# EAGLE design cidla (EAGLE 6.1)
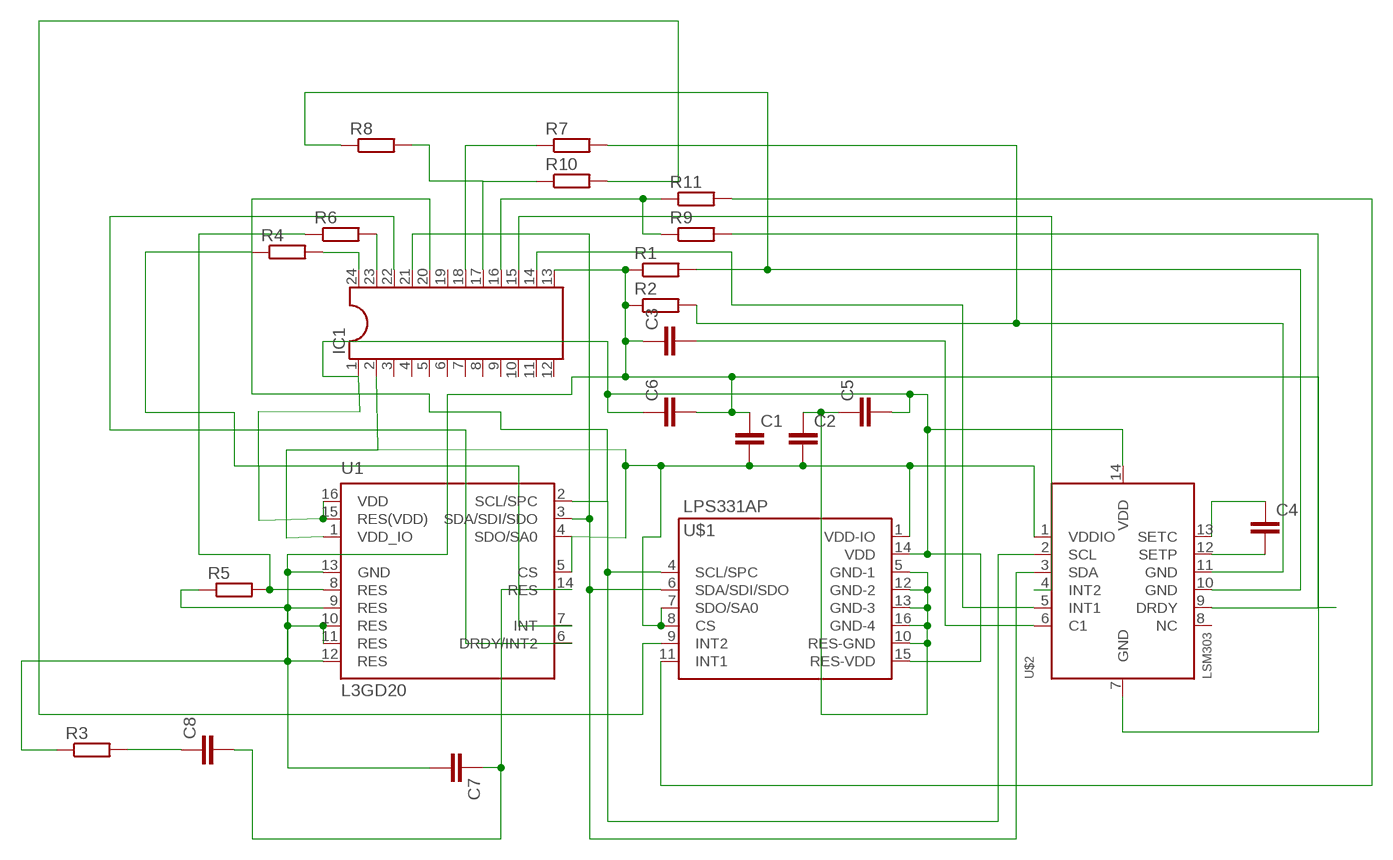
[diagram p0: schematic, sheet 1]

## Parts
C1  C-EUC0402  [C0402]
C2  C-EUC0402  [C0402]
C3  C-EUC0402  [C0402]
C4  C-EUC0402  [C0402]
C5  C-EUC0402  [C0402]
C6  C-EUC0402  [C0402]
C7  C-EUC0402  [C0402]
C8  C-EUC0402  [C0402]
IC1  DIL24-6  [DIL24-6]
R1  R-EU_R0402  [R0402]
R2  R-EU_R0402  [R0402]
R3  R-EU_R0402  [R0402]
R4  R-EU_R0402  [R0402]
R5  R-EU_R0402  [R0402]
R6  R-EU_R0402  [R0402]
R7  R-EU_R0402  [R0402]
R8  R-EU_R0402  [R0402]
R9  R-EU_R0402  [R0402]
R10  R-EU_R0402  [R0402]
R11  R-EU_R0402  [R0402]
U1  L3GD20  [LGA-16L]
U$1  LPS331AP  [HCLGA-16L]
U$2  LSM303  [LGA14]

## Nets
N$1: C5.2 C6.1 IC1.1 U1.15(RES(VDD)) U1.16(VDD) U$1.14(VDD) U$1.15(RES-VDD) U$2.14(VDD)
N$2: C1.2 C2.2 IC1.2 U1.1(VDD_IO) U1.4(SDO/SA0) U1.5(CS) U$1.1(VDD-IO) U$1.7(SDO/SA0) U$1.8(CS) U$2.1(VDDIO)
N$3: C1.1 C3.1 C6.2 C7.2 IC1.13 R1.1 R2.1 R3.1 R5.1 U1.9(RES) U1.10(RES) U1.11(RES) U1.12(RES) U1.13(GND) U$2.7(GND)
N$4: IC1.24 R4.2
N$5: IC1.23 R6.2
N$6: IC1.17 R8.2 R10.1
N$7: IC1.18 R7.1
N$8: IC1.16 R9.1 R11.1
N$9: IC1.14 U$2.5(INT1)
N$10: C3.2 U$2.6(C1)
N$12: R11.2 U$1.11(INT1)
N$14: C2.1 C5.1 U$1.5(GND-1) U$1.10(RES-GND) U$1.12(GND-2) U$1.13(GND-3) U$1.16(GND-4)
N$16: R10.2 U$1.9(INT2)
N$17: R1.2 R8.1 U$2.10(GND)
N$18: C4.2 U$2.12(SETP)
N$19: C4.1 U$2.13(SETC)
N$20: R2.2 R7.2 U$2.11(GND)
N$21: IC1.15 U$2.4(INT2)
N$22: IC1.21 U1.3(SDA/SDI/SDO) U$1.6(SDA/SDI/SDO) U$2.3(SDA)
N$23: IC1.20 U1.2(SCL/SPC) U$1.4(SCL/SPC) U$2.2(SCL)
N$24: R4.1 U1.7(INT)
N$25: C7.1 C8.2 U1.14(RES)
N$26: R5.2 R6.1 U1.8(RES)
N$27: IC1.22 U1.6(DRDY/INT2)
N$28: C8.1 R3.2
N$29: R9.2 U$2.9(DRDY)
Unconnected: IC1.3 IC1.4 IC1.5 IC1.6 IC1.7 IC1.8 IC1.9 IC1.10 IC1.11 IC1.12 IC1.19 U$2.8(NC)

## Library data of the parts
C1-C8 = rcl:C-EU: CAPACITOR, European symbol
IC1 = ic-package:DIL24: Dual In Line
R1-R11 = rcl:R-EU_: RESISTOR, European symbol
U1 = cansat_jecnaci:L3GD20: L3GD20 MEMS motion sensor - three-axis digital output gyroscope
U$1 = cansat_jecnaci:LPS331AP: LPS331AP MEMS pressure sensor: 260-1260 mbar absolute digital output barometer Features ? 260 to 1260 mbar absolute pressure range ? High-resolution mode: 0.020 mbar RMS ? Low power consumption: ? Low resolution mode: 5.5 ?A ? High resolution mode: 30 ?A ? High overpressure capability: 20x full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
U$2 = LSM303:LSM303

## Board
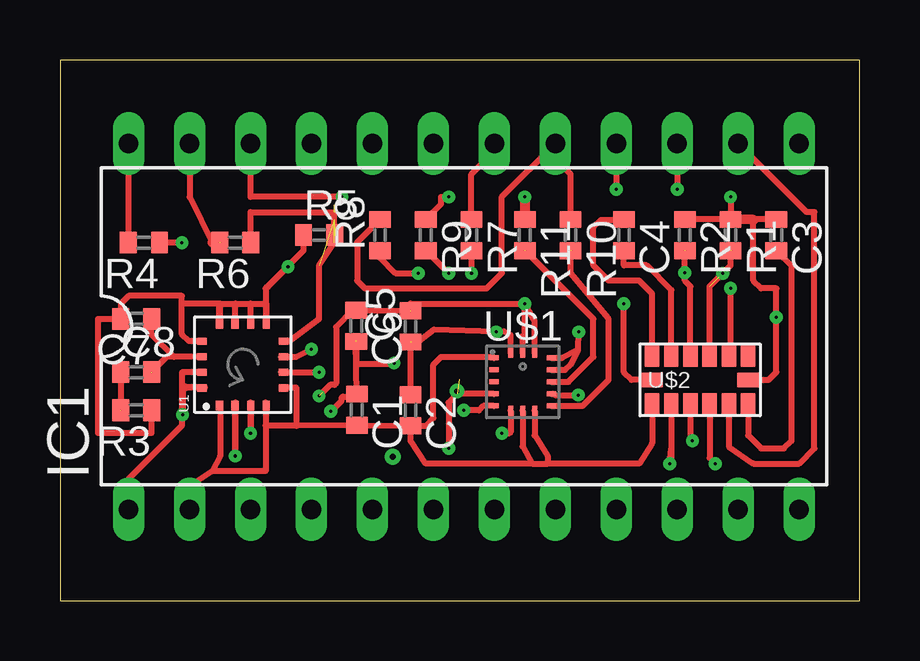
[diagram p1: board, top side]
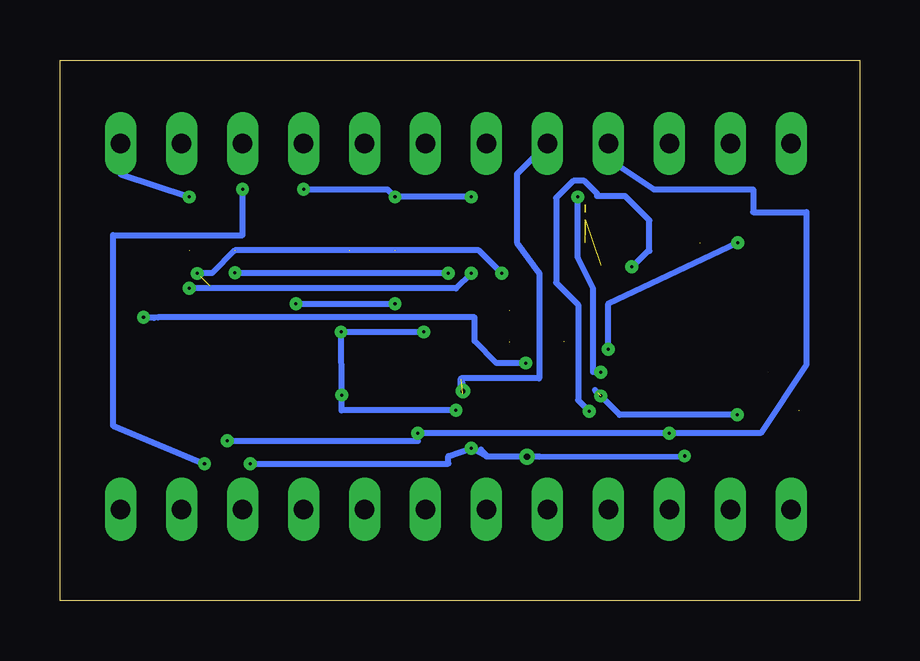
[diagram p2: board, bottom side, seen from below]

Size 33.33 x 22.53 mm. Coordinates in mm from the lower left corner, seen from the top.
Outline: 0,0 33.33,0 33.33,22.53 0,22.53 0,0
Copper layers (1*16): Top 0.035mm / dielectric 1.5mm / Bottom 0.035mm
Design rules "default": minimum track width 10mil, minimum drill 24mil, track to track 8mil, track to pad 8mil, pad to pad 8mil, via to via 8mil, smd to smd 8mil, copper to edge 40mil, drill to drill 8mil, minimum pad ring 10mil, minimum via ring 8mil, stop-mask expansion 4mil, vias tented up to drill 0mil, thermal gap 10mil

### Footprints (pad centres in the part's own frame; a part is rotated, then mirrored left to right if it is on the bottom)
C0402 = smd 0.7 x 0.9: 1 -0.65,0; 2 0.65,0
DIL24-6 = drill 0.813 long: 1 -13.97,-7.62; 2 -11.43,-7.62; 3 -8.89,-7.62; 4 -6.35,-7.62; 5 -3.81,-7.62; 6 -1.27,-7.62; 7 1.27,-7.62; 8 3.81,-7.62; 9 6.35,-7.62; 10 8.89,-7.62; 11 11.43,-7.62; 12 13.97,-7.62; 13 13.97,7.62; 14 11.43,7.62; 15 8.89,7.62; 16 6.35,7.62; 17 3.81,7.62; 18 1.27,7.62; 19 -1.27,7.62; 20 -3.81,7.62; 21 -6.35,7.62; 22 -8.89,7.62; 23 -11.43,7.62; 24 -13.97,7.62
R0402 = smd 0.7 x 0.9: 1 -0.65,0; 2 0.65,0
LGA-16L = smd 0.4 x 0.3: 1 -1.7,0.975; 2 -1.7,0.325; 3 -1.7,-0.325; 4 -1.7,-0.975; 9 1.7,-0.975; 10 1.7,-0.325; 11 1.7,0.325; 12 1.7,0.975 | smd 0.3 x 0.4: 5 -0.975,-1.7; 6 -0.325,-1.7; 7 0.325,-1.7; 8 0.975,-1.7; 13 0.975,1.7; 14 0.325,1.7; 15 -0.325,1.7; 16 -0.975,1.7
HCLGA-16L = smd 0.406 x 0.203: 1 0.3,2.5; 2 0.3,2; 3 0.3,1.5; 4 0.3,1; 5 0.3,0.5; 9 2.7,0.5; 10 2.7,1; 11 2.7,1.5; 12 2.7,2; 13 2.7,2.5 | smd 0.203 x 0.406: 6 1,0.3; 7 1.5,0.3; 8 2,0.3; 14 2,2.7; 15 1.5,2.7; 16 1,2.7
LGA14 = smd 0.9 x 0.6: 1 1,-2; 2 1,-1.2; 3 1,-0.4; 4 1,0.4; 5 1,1.2; 6 1,2; 8 -1,2; 9 -1,1.2; 10 -1,0.4; 11 -1,-0.4; 12 -1,-1.2; 13 -1,-2 | smd 0.6 x 0.9: 7 0,2; 14 0,-2

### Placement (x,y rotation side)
C1  12.37,7.96 270 top
C2  14.61,7.94 270 top
C3  29.84,15.24 270 top
C4  23.5,15.24 270 top
C5  14.61,11.43 90 top
C6  12.34,11.46 270 top
C7  3.17,11.75 180 top
C8  3.17,9.53 0 top
IC1  16.83,11.43 0 top
R1  27.94,15.24 270 top
R2  26.04,15.24 270 top
R3  3.17,7.94 180 top
R4  3.49,14.92 180 top
R5  10.79,15.24 0 top
R6  7.3,14.92 180 top
R7  17.14,15.24 270 top
R8  13.34,15.24 90 top
R9  15.24,15.24 270 top
R10  21.27,15.24 270 top
R11  19.37,15.24 270 top
U1  7.62,9.84 90 top
U$1  17.78,7.62 0 top
U$2  26.67,9.21 270 top

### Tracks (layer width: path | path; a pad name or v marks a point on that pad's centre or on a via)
N$1  (via drill 0.13)  (2 unrouted)
  Top 0.254: U1.15 5.08,9.52 5.08,9.07 | 5.08,9.07 5.08,8.89 5.11,8.89 | IC1.1 2.86,5.08 5.08,7.3 5.08,8.87 U1.16 5.28,8.87 5.08,9.07 | v19.37,12.38 14.61,12.38 14.59,12.08 C6.1 12.21,12.11 11.51,11.4 11.51,9.07 11.43,8.99 11.25,8.99 v10.79,8.53 | v19.37,12.38 19.37,11.11 19.28,11.03 U$1.15 | U$1.14 19.78,11.65 19.58,12.01 v19.37,12.38 | U$2.14 23.81,9.21 23.5,9.53 v23.5,12.38 | 6.03,8.89 5.11,8.89 | 5.11,8.89 5.11,8.91 | 5.11,8.89 v5.11,7.75
  Bottom 0.254: v23.5,12.38 v19.37,12.38 | v5.11,7.75 10.01,7.75 v10.79,8.53 10.92,8.66 11.04,8.78
N$2
  Top 0.254: U1.1 6.67,8.12 6.67,6.03 6.35,5.4 | 6.35,5.4 5.4,4.76 IC1.2 | 8.57,8.12 U1.4 8.57,8.16 | 8.57,8.12 8.57,7.3 | 8.57,7.3 8.57,5.4 6.35,5.4 | U1.5 9.34,8.89 9.84,8.89 9.84,7.3 | 9.84,7.3 8.57,7.3 | 8.57,8.12 8.57,8.16 | 8.57,8.16 8.57,8.26 | 19.68,5.71 20.32,5.71 | U$1.8 19.78,6.89 20.32,6.03 20.32,5.71 | U$2.1 24.67,6.57 24.13,5.71 20.32,5.71 | 14.61,7.3 14.59,7.29 C1.2 9.86,7.29 9.84,7.3 | 14.61,7.3 C2.2 14.61,6.67 15.24,5.71 19.68,5.71 | 14.61,7.3 15.24,7.3 15.56,7.62 15.56,9.84 15.88,10.16 18.04,10.16 U$1.1 | U$1.7 19.28,6.44 19.68,5.71
N$3  (via drill 0.13)  (1 unrouted)
  Top 0.254: 6.67,12.38 6.67,11.56 U1.12 6.64,12.36 6.67,12.38 | 6.67,12.38 7.3,12.38 | 7.3,12.38 7.94,12.38 | 7.94,12.38 8.57,12.38 | 8.57,12.38 8.6,12.36 U1.9 8.6,13.06 8.61,13.08 8.66,13.08 v9.5,13.92 | U1.10 7.94,11.55 7.94,12.38 | U1.11 7.3,11.55 7.3,12.38 | U1.13 5.38,10.82 5.08,11.11 5.08,12.38 | 5.08,12.38 5.08,12.7 2.86,12.7 2.54,12.38 2.54,11.76 C7.2 1.59,11.75 1.59,6.99 3.81,6.99 R3.1 | 6.67,12.38 5.08,12.38 | R5.1 10.14,14.59 8.57,13.02 8.57,12.38 | 12.32,10.82 C1.1 12.27,8.51 11.79,8.51 11.73,8.46 11.73,8.33 11.3,7.9 v11.28,7.9 | C3.1 R1.1 | R1.1 R2.1 | v27.94,16.83 R1.1 | U$2.7 29.53,9.21 29.84,9.53 v29.84,11.81 29.84,13.02 29.21,13.02 28.89,13.34 28.89,15.88 | C6.2 12.34,9.91 12.37,9.88 13.89,9.88 v13.92,9.91
  Top 0.406: 27.94,15.88 27.95,15.89 R1.1 28.89,15.88
  Bottom 0.254: v27.94,16.83 30.8,17.78 IC1.13 | v13.92,9.91 15.14,9.91 16.05,10.82 16.05,11.81 29.23,11.81 29.41,11.79 29.82,11.79 v29.84,11.81 | v9.5,13.92 9.47,13.92 8.81,14.58 8.76,14.58 8.76,15.85 9.78,16.87 10.95,16.87 10.95,16.97 11.48,17.5 11.94,17.5 12.65,16.79 12.65,13.26 11.73,12.34 11.73,8.36 v11.28,7.9
N$4
  Top 0.254: 2.86,14.92 IC1.24
  Top 0.406: R4.2 2.86,14.92
N$5  (1 unrouted)
  Top 0.254: IC1.23 5.4,16.83 6.35,14.92
  Top 0.406: 6.35,14.92 6.67,14.92
N$6
  Top 0.254: R10.1 21.27,17.78 20.64,18.41 IC1.17 18.41,16.83 18.41,13.65 17.78,13.02 12.7,13.02 12.38,13.34 12.38,14.94 R8.2
N$7
  Top 0.254: R7.1 17.14,17.78 18.1,18.73 IC1.18
N$8  (via drill 0.13)
  Top 0.254: R9.1 15.88,16.52 15.88,16.83 v16.19,16.83 | IC1.16 v23.18,17.14
  Top 0.406: v19.37,16.83 R11.1
  Bottom 0.254: v16.19,16.83 v19.37,16.83 19.68,17.14 v23.18,17.14
N$9
  Top 0.254: U$2.5 27.87,6.42 28.89,5.71 30.8,5.71 31.43,6.35 31.43,16.19 31.11,16.19 IC1.14
N$10
  Top 0.254: U$2.6 28.67,6.89 29.21,6.35 30.16,6.35 30.48,6.67 30.48,13.97 30.46,13.97 C3.2
N$12  (1 unrouted)
  Top 0.254: U$1.11 21.18,9.12 22.23,10.16 22.23,11.75 19.37,14.61
N$14  (via drill 0.13)  (1 unrouted)
  Top 0.254: C2.1 14.61,10.79 14.92,10.79 15.58,11.3 v18.17,11.2 18.49,11.23 18.78,11.06 U$1.16 | U$1.12 21.05,9.62 21.27,9.84 21.59,10.48 | U$1.13 20.91,10.12 21.59,10.48 | 21.59,10.48 v21.61,11.2 | U$1.10 20.64,8.57 v21.59,8.57 | U$1.5 17.64,8.12 17.46,7.94 v16.83,7.94
  Bottom 0.254: v18.17,11.2 v21.61,11.2 v21.59,8.57 21.59,7.94 v16.83,7.94
N$16  (1 unrouted)
  Top 0.254: U$1.9 21.77,8.12 22.86,9.21 22.86,11.75 21.27,13.65 21.27,14.61
N$17  (via drill 0.13)  (2 unrouted)
  Top 0.254: U$2.10 27.07,13.1 v27.61,13.64 27.94,13.97 27.94,14.61 | R8.1 13.34,14.29 13.97,13.65 v14.92,13.65
  Bottom 0.254: v14.92,13.65 15.88,14.61 26.04,14.61 26.99,13.65 27.62,13.65
N$18
  Top 0.254: U$2.12 25.47,12.95 24.45,13.97 23.5,13.97 C4.2
N$19
  Top 0.254: U$2.13 24.67,12.79 24.13,13.34 22.86,13.34 22.23,13.97 22.23,15.56 22.54,15.88 23.5,15.88 C4.1
N$20  (via drill 0.13)  (1 unrouted)
  Top 0.254: U$2.11 26.27,13.1 26.04,13.34 26.04,13.65 v26.04,13.66 26.04,14.61 | R7.2 v17.14,13.65
  Bottom 0.254: v17.14,13.65 26.04,13.65
N$21  (via drill 0.13)
  Top 0.254: U$2.4 27.07,5.95 v27.3,5.71 | IC1.15 v25.72,17.14
  Bottom 0.254: v27.3,5.71 31.11,7.3 31.11,15.24 25.72,15.24 v25.72,17.14
N$22  (via drill 0.13)
  Top 0.254: U$2.3 26.27,6.75 v26.35,6.67 | U$1.6 18.78,7.03 18.73,6.99 v18.41,6.99 | U1.3 v7.95,6.99 v7.94,6.99 7.94,8.26 U1.3
  Bottom 0.254: v26.35,6.67 18.41,6.67 v18.41,6.99 v7.94,6.99 4.13,6.99 2.22,9.84 2.22,16.19 4.45,16.19 4.45,17.14 8.57,17.14 10.48,18.41 IC1.21
N$23  (via drill 0.13, 0.25)  (2 unrouted)
  Top 0.254: U$2.2 25.47,6.35 | 25.47,6.35 25.47,5.79 v25.4,5.71 25.47,6.35 | U$1.4 16.56,8.62 16.19,8.26 v16.19,6.35 | 7.3,6.35 7.29,6.36 U1.2 7.3,8.26 v7.3,6.03
  Bottom 0.254: v25.4,5.71 17.14,5.71 17.14,6.03 v16.19,6.35 15.56,6.03 v13.87,6.01 | v7.3,6.03 13.35,6.01 v13.87,6.01 | IC1.20 14.29,17.78 14.29,14.92 13.37,13.68 13.36,13.68 13.36,9.27 16.61,9.27 16.61,9.12 16.56,9.06 16.56,8.62 16.64,8.7 16.64,9.22 | v13.87,6.01 15.54,6.01 15.54,6.02 15.52,6.02 15.77,6.27 15.77,6.3
N$24  (via drill 0.13)
  Top 0.254: v5.08,14.92 R4.1 4.13,14.92 | v10.48,10.48 9.84,10.16 9.21,10.16 U1.7
  Bottom 0.254: v5.08,14.92 10.48,12.38 v10.48,10.48
N$25  (1 unrouted)
  Top 0.254: U1.14 4.75,10.17 | 4.75,10.17 3.81,11.11 3.81,11.73 C7.1 | 4.75,10.17 4.45,10.17 C8.2
N$26  (5 unrouted)
  Top 0.254: U1.8 9.55,10.82 10.79,11.75 10.79,13.97 11.43,14.92 11.43,16.19 7.94,16.19 7.95,16.18 R6.1
N$27  (via drill 0.13, 0.6)
  Top 0.254: v10.79,9.53 9.21,9.53 U1.6 | IC1.22 7.94,16.83 v11.75,16.83
  Bottom 0.254: v10.79,9.53 11.11,9.53 11.11,13.02 11.75,14.29 v11.75,16.83
  other vias: 7.94,19.05
N$28  (1 unrouted)
  Top 0.254: C8.1 2.52,7.95 2.54,7.94
N$29  (via drill 0.13)
  Top 0.254: R9.2 15.26,14.59 v16.19,13.65 | U$2.9 27.94,10.21 v27.94,13.02
  Bottom 0.254: v16.19,13.65 16.83,13.02 v27.94,13.02
S$1  (via drill 0.2 pad 0.25)
  other vias: 16.54,8.74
